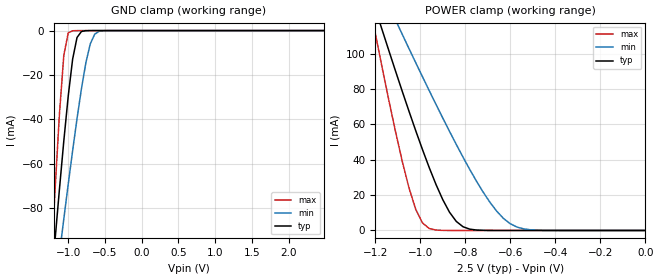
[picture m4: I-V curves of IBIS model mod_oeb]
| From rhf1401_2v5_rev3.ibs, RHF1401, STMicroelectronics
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|   Model mod_oeb
[Model]   mod_oeb
Model_type Input
Vinl   =   0.625V
Vinh   =   1.875V
C_comp   0.352pF   0.339pF   0.368pF
[Temperature Range]  27.0000   0.1250k   -55.0000
[Voltage Range]   2.5000V   2.3000V   2.7000V
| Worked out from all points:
|   GND clamp passes 1 mA (typ) near -0.83 V on its own axis
|   POWER clamp passes 1 mA (typ) near -0.79 V on its own axis
[GND_clamp]
|Voltage   I(typ)   I(min)   I(max)
-2.5V     -647mA     -491mA     -992.2mA
-1.24V    -118.3mA   -133.4mA   -110.2mA
-1.18V    -94.73mA   -117.1mA   -72.47mA
-1.12V    -71.78mA   -100.9mA   -37.89mA
-1.06V    -49.81mA   -84.98mA   -11.18mA
-1V       -29.61mA   -69.38mA   -1.046mA
-940mV    -12.92mA   -54.22mA   -82.43uA
-880mV    -3.113mA   -39.73mA   -10.57uA
-760mV    -46.21uA   -14.61mA   -27.16nA
-700mV    -4.665uA   -6.035mA   -1.125nA
-580mV    -45.36nA   -350.1uA   -8.653pA
2.48V     14.49pA    -4.639pA   14.16pA
[POWER_clamp]
|Voltage   I(typ)   I(min)   I(max)
-2.49V    667.8mA    510.6mA    1.016A
-1.23V    137.7mA    152mA      131.4mA
-1.2V     125.7mA    143.7mA    111.8mA
-1.17V    113.8mA    135.5mA    92.69mA
-1.11V    90.3mA     119.1mA    56.09mA
-1.05V    67.48mA    102.9mA    24.14mA
-990mV    45.76mA    86.97mA    4.273mA
-900mV    17.47mA    63.64mA    48.56uA
-810mV    2.109mA    41.47mA    406nA
-660mV    7.7uA      10.86mA    158.5pA
-570mV    237.5nA    1.911mA    20.1pA
0V        14.61pA    65.38pA    15.5pA
